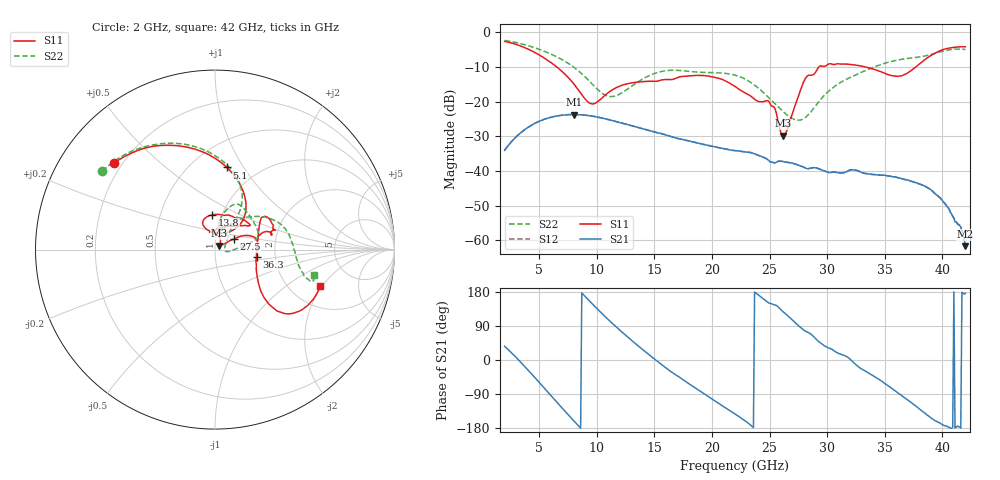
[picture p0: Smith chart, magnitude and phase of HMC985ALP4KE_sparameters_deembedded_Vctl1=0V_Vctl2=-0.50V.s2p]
!s2p File: Measurements: S11, S21, S12, S22
# GHz S dB R 50.0
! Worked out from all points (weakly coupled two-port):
!   401 points, 2 GHz to 42 GHz, reference 50 ohm
!   highest |S21| = -23.69 dB at 8 GHz (marker M1); lowest = -61.7 dB at 42 GHz (marker M2)
!   lowest |S11| = -29.8 dB at 26.2 GHz (marker M3), VSWR 1.07, Z = 52.5 + j2.23 ohm
!   |S11| at or under -10 dB: 6.535 GHz to 29.27 GHz (22.74 GHz wide, 127 % of centre); 33.34 GHz to 37.69 GHz (4.348 GHz wide, 12.2 % of centre)
!   |S22| runs from -25.4 to -2.3 dB; largest |S21 - S12| = 0.00012
!   S11 on the Smith chart (normalised r, x): 2 GHz: 0.17, +0.36; 5.1 GHz: 0.73, +0.85; 13.8 GHz: 0.90, +0.36; 27.5 GHz: 1.22, +0.15; 36.3 GHz: 1.59, -0.14; 42 GHz: 2.91, -1.91
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2  -2.60 139.7  -34.02 36.2  -34.02 36.1  -2.33 145.2
3.5  -4.08 111.8  -28.68 -9.1  -28.69 -9.2  -3.34 121.2
5.1  -6.70 81.8  -25.50 -62.3  -25.51 -62.3  -5.01 96.8
8  -14.84 45.1  -23.69 -160.3  -23.70 -160.3  -10.03 61.3
8.7  -17.98 51.6  -23.78 176.9  -23.79 176.9  -11.95 57.1
9.7  -20.63 86.7  -24.20 145.3  -24.20 145.4  -15.23 57.1
11.1  -17.13 115.4  -25.22 103.7  -25.23 103.7  -18.50 72.1
13.8  -14.26 95.2  -27.61 32.1  -27.61 32.1  -13.81 77.1
15.4  -13.94 73.0  -29.03 -6.3  -29.04 -6.3  -11.45 68.3
19.4  -12.52 34.7  -32.40 -90.9  -32.40 -91.0  -11.58 35.0
22  -15.58 52.2  -34.08 -142.2  -34.10 -142.2  -12.34 14.9
25  -20.22 97.7  -37.20 149.7  -37.21 149.6  -19.08 0.7
26.2  -29.80 41.1  -37.25 126.8  -37.26 126.7  -22.91 -9.1
27.5  -18.42 29.6  -38.26 91.1  -38.30 90.8  -25.31 1.4
28.1  -13.37 20.7  -39.09 76.3  -39.08 76.3  -24.58 18.6
28.7  -12.32 12.8  -39.06 65.5  -39.11 65.4  -22.45 33.8
31  -9.09 23.4  -40.51 17.1  -40.55 17.3  -14.76 53.3
35.4  -12.27 12.4  -41.43 -70.4  -41.47 -70.7  -8.56 25.2
36.3  -12.57 -10.1  -42.02 -90.2  -42.07 -90.5  -7.88 17.6
39.8  -5.31 -41.3  -47.79 -166.2  -47.60 -167.4  -5.62 -16.5
41.5  -4.18 -23.0  -55.74 -176.5  -55.48 -176.8  -4.79 -17.2
42  -4.14 -19.0  -61.66 175.7  -61.52 172.8  -4.93 -14.2
